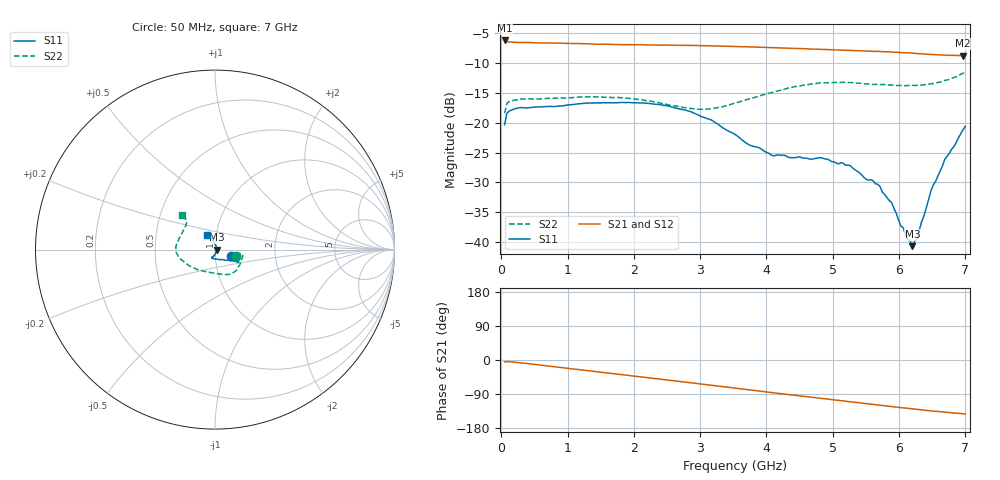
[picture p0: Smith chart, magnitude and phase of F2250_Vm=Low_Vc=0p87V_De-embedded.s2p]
! Integrated Device Technology
! Corporate Headquarters
! 6024 Silver Creek Valley Road
! San Jose, CA 95138  USA
! Phone:  1-408-284-8200
! Toll Free:  1-800-223-1366
! Webpage:  http://www.idt.com/
! Timing and RF Division
! 515 Groton Road, Suite 102
! Westford, MA 01886-6024
! Device:  F2250
! Description: Voltage Variable RF Attenuator
! Frequency:  50.0 -  6000.00 MHz
! Package:  3x3 mm Thin QFN Plastic Package: 16 pin
! Ports:  2 RF, 3 DC
!  Pin  1  = GND
!  Pin  2  = NC
!  Pin  3  = RF1  = Port 1
!  Pin  4  = NC
!  Pin  5  = GND
!  Pin  6  = GND
!  Pin  7  = GND
!  Pin  8  = GND
!  Pin  9  = NC
!  Pin 10  = RF2  = Port 2
!  Pin 11  = NC
!  Pin 12  = GND
!  Pin 13  = GND
!  Pin 14  = VCNTRL
!  Pin 15  = VDD
!  Pin 16  = VMODE
! Vcntrl:  0.870 Volts
! Vmode:  +0.000 Volts
! Vdd:  +3.30  Volts
! Current:  1.173 mA
! Data:  The device was measured on a the F2250 evaluation board which has
!  individual transmission lines to the RF pins.  Data was collected
!  using a calibrated network analyzer.  The evaluation board was
!  de-embedded using a TRL calibration technique.
!  The reference plane is the edge of the package pin.
! Misc:  SN 10
!  Action Tracker AT0258
! Date Measured:  2014-11-26
! Date:  2015-10-15  MJV
! Note:
!  Integrated Device Technology supplies this data as a sample of measured
!  data at the package pin for this product.  Your particular data for this
!  product may vary.
!  Data was taken at 25 degrees C.
!  Integrated Device Technology reserves the right to change this data at anytime.
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# GHz S dB R 50
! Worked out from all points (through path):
!   201 points, 50 MHz to 7 GHz, reference 50 ohm
!   highest |S21| = -6.17 dB at 50 MHz (marker M1); lowest = -8.7 dB at 6.965 GHz (marker M2)
!   group delay of S21, straight-line fit = 57 ps
!   lowest |S11| = -40.7 dB at 6.201 GHz (marker M3), VSWR 1.02, Z = 50.9 + j0.00123 ohm
!   |S11| at or under -10 dB: start of sweep to end of sweep
!   |S22| runs from -18.4 to -11.5 dB; largest |S21 - S12| = 0.0015
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0.05  -20.30 -21.4  -6.17 -5.3  -6.16 -5.3  -18.37 -16.3
0.08475  -18.39 -11.0  -6.35 -4.5  -6.36 -4.5  -16.71 -9.4
0.22375  -17.57 -8.0  -6.49 -6.1  -6.49 -6.1  -16.15 -10.6
1.2315  -16.74 -24.9  -6.72 -26.7  -6.71 -26.7  -15.63 -42.5
2.37825  -16.91 -28.9  -6.93 -50.0  -6.93 -50.0  -16.62 -70.1
3.0385  -19.02 -33.6  -7.04 -63.9  -7.04 -63.9  -17.74 -101.1
3.525  -21.92 -46.9  -7.18 -74.2  -7.17 -74.2  -16.68 -129.8
4.081  -25.46 -79.0  -7.36 -86.0  -7.36 -86.0  -14.91 -155.2
4.7065  -26.03 -109.7  -7.62 -99.0  -7.63 -99.0  -13.46 -173.1
4.81075  -25.83 -110.6  -7.66 -101.1  -7.66 -101.2  -13.30 -175.2
5.2625  -27.17 -107.5  -7.83 -110.4  -7.84 -110.4  -13.23 174.3
5.50575  -29.47 -99.7  -7.95 -115.3  -7.95 -115.3  -13.46 168.4
5.6795  -30.31 -92.9  -8.00 -118.8  -8.00 -118.8  -13.55 163.8
5.85325  -33.05 -81.9  -8.08 -122.2  -8.11 -122.3  -13.64 159.3
5.888  -33.37 -80.3  -8.12 -123.0  -8.14 -122.9  -13.64 158.7
6.027  -37.32 -62.8  -8.21 -125.7  -8.22 -125.7  -13.73 154.0
6.20075  -40.69 0.1  -8.32 -129.2  -8.31 -129.2  -13.70 148.2
6.27025  -39.49 35.6  -8.35 -130.5  -8.36 -130.5  -13.70 146.0
6.5135  -30.46 87.2  -8.54 -134.8  -8.53 -134.8  -13.42 138.5
6.68725  -26.16 100.1  -8.63 -137.6  -8.66 -137.6  -12.89 134.6
6.96525  -21.15 118.4  -8.70 -142.0  -8.70 -142.0  -11.68 133.7
7  -20.57 119.7  -8.69 -142.5  -8.71 -142.5  -11.48 133.2
